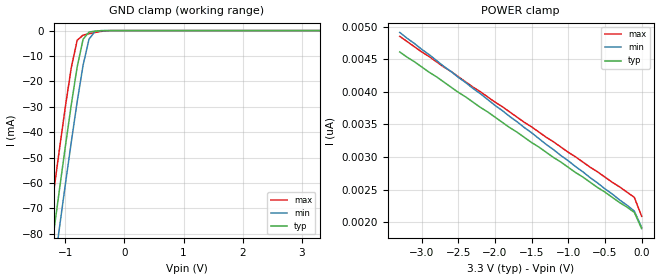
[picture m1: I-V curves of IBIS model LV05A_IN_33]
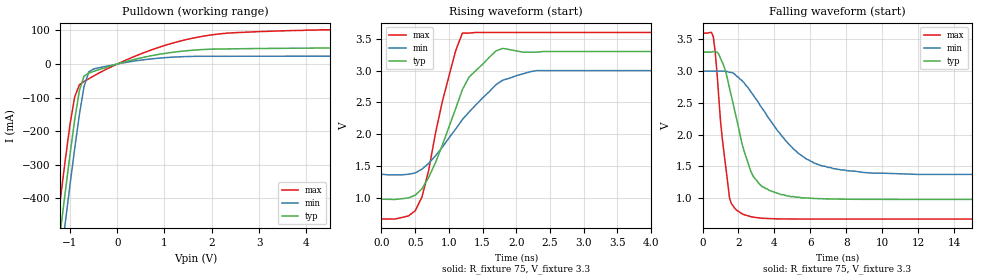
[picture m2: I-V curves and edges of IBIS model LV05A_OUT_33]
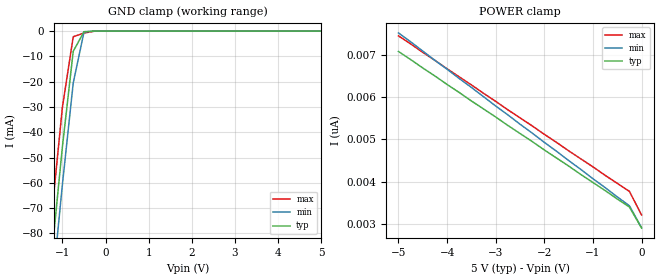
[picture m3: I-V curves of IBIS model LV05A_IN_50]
| TEXAS INSTRUMENTS INCORPORATED
| Standard Linear and Logic Group
| IBIS Model of SN74LV05A
| HEX INVERTER WITH OPEN-DRAIN OUTPUTS
| SOIC 14-pin (D), SOP 14-pin (NS), SSOP 14-pin (DB), TSSOP 14-pin (PW)
| and TVSOP 14-pin (DGV) Package
[IBIS Ver]   3.2
[Comment Char]  |_char
[File Name]   lv05a.ibs
[File Rev]   2.0 I_die
[Date]   May 24, 2000
[Source]   Data created from HSPICE simulations at TI-SLL.
[Notes]   The following is an IBIS list for the LV05A.
|   Please contact sllibis@ti.com with questions and
|   comments concerning SLL IBIS models.
[Disclaimer] Property of Texas Instruments Incorporated.  Unauthorized
   reproduction and/or distribution is strictly prohibited.
   This product is protected under copyright law.
   Created 2000, (C) Copyright 2000, Texas Instruments Inc.,
   All Rights Reserved.
   UNLESS THERE IS A SIGNED, WRITTEN AGREEMENT TO THE
   CONTRARY, TEXAS INSTRUMENTS () IS PROVIDING THE IBIS
   MODELS  AND WITHOUT ANY WARRANTY, EXPRESSED OR
   IMPLIED.  TI assumes no liability for:
   1) the accuracy of the IBIS models provided to your
   company;
   2) the proper functioning of these IBIS Models in your
   design or for any resulting applications; or
   3) infringement of patents, copyrights or intellectual
   property rights resulting from your use of these IBIS
   models.
   TI provides IBIS Models as a service to our customers.
   You and your company shall not distribute, sell or give
   these models to anyone else without prior written
   permission from TI.
   TI reserves the right to make changes to our products or
   to discontinue any semiconductor product or service
   without notice, and advises our customers to obtain the
   latest version of relevant information to verify, before
   placing orders, that the information being relied on is
   current.
   Please be aware that your receipt and use of the IBIS
   information provided shall serve as acceptance of these
   terms and conditions.  If you do not accept these terms,
   you should return or destroy the IBIS models and any
   other accompanying information immediately.
|   Component LV05A_D
[Component]   LV05A_D
[Manufacturer]  Texas Instruments, Inc.
[Package]
|   typ   min   max
R_pkg   0.031   0.028   0.034
L_pkg   3.109nH   2.462nH   3.889nH
C_pkg   0.473pF   0.363pF   0.628pF
[Pin]   signal_name   model_name   R_pin   L_pin   C_pin
1   1A   LV05A_IN   0.033   3.854nH   0.622pF
2   1Y   LV05A_OUT   0.032   3.188nH   0.473pF
3   2A   LV05A_IN   0.028   2.462nH   0.377pF
4   2B   LV05A_OUT   0.031   2.596nH   0.363pF
5   3A   LV05A_IN   0.028   2.521nH   0.372pF
6   3Y   LV05A_OUT   0.034   3.250nH   0.476pF
7   GND   GND   0.034   3.889nH   0.628pF
8   4Y   LV05A_OUT   0.034   3.889nH   0.628pF
9   4A   LV05A_IN   0.034   3.250nH   0.476pF
10   5Y   LV05A_OUT   0.028   2.521nH   0.372pF
11   5A   LV05A_IN   0.031   2.596nH   0.364pF
12   6Y   LV05A_OUT   0.028   2.462nH   0.377pF
13   6A   LV05A_IN   0.032   3.188nH   0.473pF
14   VCC   POWER   0.033   3.854nH   0.622pF
|   Component LV05A_NS
[Component]   LV05A_NS
[Manufacturer]  Texas Instruments, Inc.
[Package]
|   typ   min   max
R_pkg   0.045   0.039   0.054
L_pkg   3.796nH   2.561nH   4.952nH
C_pkg   0.528pF   0.288pF   0.710pF
[Pin]   signal_name   model_name   R_pin   L_pin   C_pin
1   1A   LV05A_IN   0.047   4.867nH   0.706pF
2   1Y   LV05A_OUT   0.051   4.083nH   0.592pF
3   2A   LV05A_IN   0.041   2.915nH   0.376pF
4   2Y   LV05A_OUT   0.039   2.561nH   0.288pF
5   3A   LV05A_IN   0.041   3.101nH   0.430pF
6   3Y   LV05A_OUT   0.047   4.047nH   0.589pF
7   GND   GND   0.051   4.909nH   0.700pF
8   4Y   LV05A_OUT   0.045   4.784nH   0.694pF
9   4A   LV05A_IN   0.054   4.176nH   0.597pF
10   5Y   LV05A_OUT   0.039   3.287nH   0.449pF
11   5A   LV05A_IN   0.039   2.586nH   0.294pF
12   6Y   LV05A_OUT   0.040   2.802nH   0.371pF
13   6A   LV05A_IN   0.049   4.080nH   0.593pF
14   VCC   POWER   0.052   4.952nH   0.710pF
|   Component LV05A_DB
[Component]   LV05A_DB
[Manufacturer]  Texas Instruments, Inc.
[Package]
|   typ   min   max
R_pkg   0.044   0.041   0.046
L_pkg   3.551nH   3.258nH   3.927nH
C_pkg   0.402pF   0.360pF   0.421pF
[Pin]   signal_name   model_name   R_pin   L_pin   C_pin
1   1A   LV05A_IN   0.046   3.927nH   0.408pF
2   1Y   LV05A_OUT   0.044   3.587nH   0.421pF
3   2A   LV05A_IN   0.041   3.289nH   0.398pF
4   2Y   LV05A_OUT   0.042   3.258nH   0.360pF
5   3A   LV05A_IN   0.041   3.286nH   0.403pF
6   3Y   LV05A_OUT   0.044   3.586nH   0.421pF
7   GND   GND   0.046   3.927nH   0.408pF
8   4Y   LV05A_OUT   0.046   3.927nH   0.408pF
9   4A   LV05A_IN   0.044   3.586nH   0.421pF
10   5Y   LV05A_OUT   0.041   3.286nH   0.403pF
11   5A   LV05A_IN   0.043   3.258nH   0.360pF
12   6Y   LV05A_OUT   0.041   3.289nH   0.398pF
13   6A   LV05A_IN   0.044   3.587nH   0.421pF
14   VCC   POWER   0.046   3.927nH   0.408pF
|   Component LV05A_PW
[Component]   LV05A_PW
[Manufacturer]  Texas Instruments, Inc.
[Package]
|   typ   min   max
R_pkg   0.032   0.029   0.035
L_pkg   2.378nH   2.170nH   2.680nH
C_pkg   0.314pF   0.270pF   0.335pF
[Pin]   signal_name   model_name   R_pin   L_pin   C_pin
1   1A   LV05A_IN   0.033   2.618nH   0.330pF
2   1Y   LV05A_OUT   0.031   2.313nH   0.317pF
3   2A   LV05A_IN   0.030   2.310nH   0.314pF
4   2Y   LV05A_OUT   0.031   2.173nH   0.272pF
5   3A   LV05A_IN   0.030   2.204nH   0.309pF
6   3Y   LV05A_OUT   0.032   2.315nH   0.317pF
7   GND   GND   0.035   2.680nH   0.335pF
8   4Y   LV05A_OUT   0.033   2.640nH   0.333pF
9   4A   LV05A_IN   0.034   2.347nH   0.319pF
10   5Y   LV05A_OUT   0.029   2.277nH   0.313pF
11   5A   LV05A_IN   0.031   2.170nH   0.270pF
12   6Y   LV05A_OUT   0.031   2.244nH   0.311pF
13   6A   LV05A_IN   0.033   2.343nH   0.321pF
14   VCC   POWER   0.035   2.657nH   0.332pF
|   Component LV05A_DGV
[Component]   LV05A_DGV
[Manufacturer]  Texas Instruments, Inc.
[Package]
|   typ   min   max
R_pkg   0.035   0.020   0.045
L_pkg   2.499nH   2.077nH   2.966nH
C_pkg   0.361pF   0.305pF   0.416pF
[Pin]   signal_name   model_name   R_pin   L_pin   C_pin
1   1A   LV05A_IN   0.027   2.717nH   0.373pF
2   1Y   LV05A_OUT   0.037   2.434nH   0.398pF
3   2A   LV05A_IN   0.034   2.200nH   0.316pF
4   2Y   LV05A_OUT   0.020   2.077nH   0.309pF
5   3A   LV05A_IN   0.030   2.147nH   0.305pF
6   3Y   LV05A_OUT   0.042   2.580nH   0.408pF
7   GND   GND   0.039   2.921nH   0.385pF
8   4Y   LV05A_OUT   0.033   2.841nH   0.380pF
9   4A   LV05A_IN   0.042   2.611nH   0.410pF
10   5Y   LV05A_OUT   0.038   2.331nH   0.329pF
11   5A   LV05A_IN   0.026   2.223nH   0.319pF
12   6Y   LV05A_OUT   0.034   2.259nH   0.313pF
13   6A   LV05A_IN   0.045   2.681nH   0.416pF
14   VCC   POWER   0.042   2.966nH   0.386pF
[Model Selector]   LV05A_IN
LV05A_IN_33   3.3-V Vcc Input Model
LV05A_IN_50   5.0-V Vcc Input Model
[Model Selector]   LV05A_OUT
LV05A_OUT_33   3.3-V Vcc Output Model
LV05A_OUT_50   5.0-V Vcc Output Model
| Models and submodels in the file (4): LV05A_IN_33 (Input), LV05A_OUT_33 (Open_drain), LV05A_IN_50 (Input), LV05A_OUT_50 (Open_drain)
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|   Model LV05A_IN_33
[Model]   LV05A_IN_33
Model_type  Input
Polarity   Inverting
Vinl = 0.99
Vinh = 2.31
| variable   typ   min   max
C_comp   1.24pf   0.94pf   1.54pf
[Temperature Range]   25   85   -40
[Voltage Range]   3.3   3.0   3.6
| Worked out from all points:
|   GND clamp passes 1 mA (typ) near -0.61 V on its own axis
[GND Clamp]
|   Voltage   I(typ)   I(min)   I(max)
-3.3V     -460mA     -475mA     -445mA
-1.3V     -97.5mA    -113mA     -81.5mA
-1.2V     -79.9mA    -95mA      -63.9mA
-1.1V     -62.6mA    -77.6mA    -46.7mA
-1V       -45.6mA    -60.5mA    -30mA
-900mV    -29.2mA    -43.9mA    -14.6mA
-800mV    -14.3mA    -28mA      -3.81mA
-700mV    -3.42mA    -13.6mA    -1.78mA
-600mV    -581uA     -3.4mA     -1.25mA
-500mV    -233uA     -353uA     -759uA
-400mV    -58.1uA    -21.9uA    -324uA
3.3V      1.9nA      2.34nA     1.69nA
[POWER Clamp]
|   Voltage   I(typ)   I(min)   I(max)
-3.3V     4.61nA     4.91nA     4.85nA
-3V       4.38nA     4.65nA     4.61nA
-100mV    2.15nA     2.17nA     2.38nA
0V        1.9nA      1.92nA     2.09nA
|   Model LV05A_OUT_33
[Model]   LV05A_OUT_33
Model_type  Open_drain
Polarity   Non-Inverting
Vmeas = 1.65v
Cref = 15pf
| variable   typ   min   max
C_comp   3.34pf   2.50pf   4.18pf
[Temperature Range]   25   85   -40
[Voltage Range]   3.3   3.0   3.6
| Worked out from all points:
|   slope of the pulldown table from 0 to 0.495 V, typ, clamps not added: 27.3 ohm
|   rising waveform, R_fixture 75, V_fixture 3.3: 20-80 % time 515ps typ, 776ps min, 368ps max; typ from 0.976 V to 3.3 V
|   falling waveform, R_fixture 75, V_fixture 3.3: 20-80 % time 1.24ns typ, 2.68ns min, 602ps max; typ from 3.3 V to 0.976 V
[Pulldown]
|   Voltage   I(typ)   I(min)   I(max)
-3.3V     -3.04A     -3.13A     -2.95A
-1.3V     -615mA     -707mA     -518mA
-1.2V     -498mA     -591mA     -401mA
-1.1V     -383mA     -475mA     -288mA
-900mV    -167mA     -253mA     -98.6mA
-800mV    -79.1mA    -151mA     -61.7mA
-700mV    -35.5mA    -66.4mA    -51.9mA
-600mV    -26.8mA    -23.2mA    -43.9mA
-500mV    -22mA      -14.7mA    -35.8mA
700mV     24.2mA     15mA       40.9mA
2V        44.3mA     23.1mA     86.9mA
6.6V      48.1mA     23.5mA     103mA
[Ramp]
| variable   typ   min   max
dV/dt_r   1.32E-02/2.55E-10   8.10E-03/7.23E-10   2.09E-02/1.34E-10
dV/dt_f   1.40E+00/1.20E-09   9.84E-01/2.69E-09   1.77E+00/5.22E-10
R_load = 75
[Rising Waveform]
R_fixture = 75
V_fixture = 3.3
V_fixture_min = 3.0
V_fixture_max = 3.6
|   Time   V(typ)   V(min)   V(max)
0s        976mV      1.37V      666mV
400ps     997mV      1.37V      714mV
600ps     1.14V      1.45V      1.01V
900ps     1.82V      1.79V      2.5V
1.1ns     2.4V       2.08V      3.31V
1.2ns     2.7V       2.23V      3.59V
1.3ns     2.9V       2.35V      3.59V
1.7ns     3.31V      2.78V      3.6V
2.3ns     3.29V      3V         3.6V
25ns      3.3V       3V         3.6V
[Falling Waveform]
R_fixture = 75
V_fixture = 3.3
V_fixture_min = 3.0
V_fixture_max = 3.6
|   Time   V(typ)   V(min)   V(max)
0s        3.3V       3V         3.6V
600ps     3.31V      3V         3.54V
800ps     3.3V       3V         2.99V
1ns       3.2V       3V         2.21V
1.5ns     2.73V      2.98V      1V
2.3ns     1.75V      2.82V      736mV
3.3ns     1.18V      2.42V      680mV
5.3ns     1.01V      1.71V      667mV
7.3ns     982mV      1.46V      666mV
25ns      976mV      1.37V      666mV
|   Model LV05A_IN_50
[Model]   LV05A_IN_50
Model_type  Input
Polarity   Inverting
Vinl = 1.5
Vinh = 3.5
| variable   typ   min   max
C_comp   1.24pf   0.94pf   1.54pf
[Temperature Range]   25   85   -40
[Voltage Range]   5.0   4.5   5.5
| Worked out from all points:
|   GND clamp passes 1 mA (typ) near -0.52 V on its own axis
[GND Clamp]
|   Voltage   I(typ)   I(min)   I(max)
-5V       -773mA     -786mA     -758mA
-1.5V     -133mA     -148mA     -117mA
-1.25V    -88.7mA    -104mA     -72.7mA
-1V       -45.6mA    -60.5mA    -30mA
-750mV    -7.99mA    -20.5mA    -2.23mA
-500mV    -233uA     -353uA     -759uA
-250mV    -2.63nA    -182nA     -26.9uA
5V        2.9nA      3.64nA     2.54nA
[POWER Clamp]
|   Voltage   I(typ)   I(min)   I(max)
-5V       7.08nA     7.52nA     7.45nA
-1.5V     4.37nA     4.5nA      4.73nA
-250mV    3.4nA      3.43nA     3.77nA
0V        2.9nA      2.91nA     3.21nA
